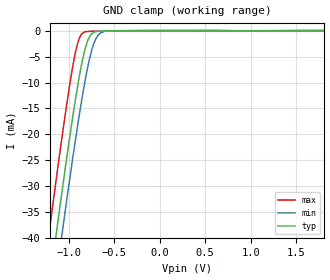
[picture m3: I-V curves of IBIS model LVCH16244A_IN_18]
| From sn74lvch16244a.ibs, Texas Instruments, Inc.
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[Model]   LVCH16244A_IN_18
Model_type  Input
Vinl=0.5775
Vinh=1.2675
| variable   typ   min   max
C_comp   3.11pF   2.47pF   4.17pF
[Temperature Range]   40   100   -40
| Ambient temperature   25   85   -40
[Voltage range]   1.8   1.65   1.95
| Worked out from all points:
|   GND clamp passes 1 mA (typ) near -0.76 V on its own axis
[GND Clamp]
| LVCH16244A_IN_18
|   Voltage   I(typ)   I(min)   I(max)
-5V       -584.6mA   -591.4mA   -576.2mA
-1.21V    -49.09mA   -57.32mA   -38.55mA
-1.135V   -39.22mA   -47.45mA   -28.66mA
-1.075V   -31.48mA   -39.69mA   -20.98mA
-1.06V    -29.58mA   -37.77mA   -19.1mA
-960mV    -17.38mA   -25.34mA   -7.567mA
-885mV    -9.203mA   -16.61mA   -1.655mA
-830mV    -4.377mA   -10.81mA   -323.7uA
-780mV    -1.559mA   -6.278mA   -154uA
-715mV    -281.3uA   -2.172mA   -118.8uA
-650mV    -86.38uA   -481.1uA   -100.5uA
1.8V      5.126pA    37.58nA    -53.97pA
